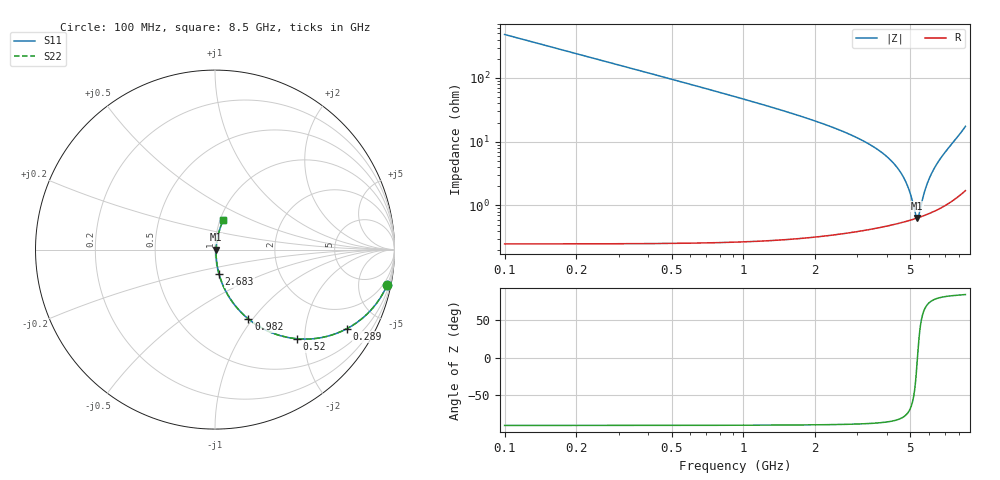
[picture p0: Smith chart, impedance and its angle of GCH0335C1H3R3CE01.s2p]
!Murata Part Number: GCH0335C1H3R3CE01
!These Parameters are Measured in Series Mode Connection
!Data Generated on Mar 13, 2026
!  o--ll--o
!Port1  Port2
!  o------o
!Operation Temp=25[degC], DC Bias Voltage=0[V]
!Freq. Start=100[MHz] Stop=9[GHz] 401[Steps]
# Hz S RI R 50
!Freq.(Hz) S11(Real) S11(Imag) S21(Real) S21(Imag) S12(Real) S12(Imag) S22(Real) S22(Imag)
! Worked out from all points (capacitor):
!   401 points, 100 MHz to 8.5 GHz, reference 50 ohm
!   read as one part in series: C = 3.3 pF near 142 MHz
!   lowest |Z| = 635 mohm at 5.35 GHz (marker M1)
!   series resonance near 5.354 GHz, so ESL is about 270 pH
!   S11 on the Smith chart (normalised r, x): 100 MHz: 1.00, -9.64; 289 MHz: 1.00, -3.33; 520 MHz: 1.01, -1.84; 982 MHz: 1.01, -0.95; 2.683 GHz: 1.01, -0.28; 8.5 GHz: 1.03, +0.35
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1e8  0.9587 -0.1988  0.0413 0.1988  0.0413 0.1988  0.9587 -0.1988
2.05e8  0.8464 -0.3601  0.1536 0.3601  0.1536 0.3601  0.8464 -0.3601
2.89e8  0.7345 -0.4409  0.2655 0.4409  0.2655 0.4409  0.7345 -0.4409
3.94e8  0.5972 -0.4894  0.4028 0.4894  0.4028 0.4894  0.5972 -0.4894
5.2e8  0.4583 -0.4969  0.5417 0.4969  0.5417 0.4969  0.4583 -0.4969
7.3e8  0.2976 -0.4552  0.7024 0.4552  0.7024 0.4552  0.2976 -0.4552
9.82e8  0.1863 -0.3866  0.8137 0.3866  0.8137 0.3866  0.1863 -0.3866
1.507e9  0.0834 -0.2717  0.9166 0.2717  0.9166 0.2717  0.0834 -0.2717
2.683e9  0.0223 -0.1352  0.9777 0.1352  0.9777 0.1352  0.0223 -0.1352
2.914e9  0.018 -0.1182  0.982 0.1182  0.982 0.1182  0.018 -0.1182
3.733e9  0.0094 -0.0698  0.9906 0.0698  0.9906 0.0698  0.0094 -0.0698
4.3e9  0.00689 -0.043  0.9931 0.043  0.9931 0.043  0.00689 -0.043
4.825e9  0.00605 -0.0209  0.994 0.0209  0.994 0.0209  0.00605 -0.0209
5.035e9  0.00603 -0.0125  0.994 0.0125  0.994 0.0125  0.00603 -0.0125
5.266e9  0.0062 -0.00341  0.9938 0.00341  0.9938 0.00341  0.0062 -0.00341
5.35e9  0.00631 -0.000148  0.9937 0.000148  0.9937 0.000148  0.00631 -0.000148
5.434e9  0.00645 0.00311  0.9936 -0.00311  0.9936 -0.00311  0.00645 0.00311
5.707e9  0.00707 0.0136  0.9929 -0.0136  0.9929 -0.0136  0.00707 0.0136
5.938e9  0.0078 0.0226  0.9922 -0.0226  0.9922 -0.0226  0.0078 0.0226
6.253e9  0.00916 0.035  0.9908 -0.035  0.9908 -0.035  0.00916 0.035
7.114e9  0.0155 0.0718  0.9845 -0.0718  0.9845 -0.0718  0.0155 0.0718
8.5e9  0.0445 0.1628  0.9555 -0.1628  0.9555 -0.1628  0.0445 0.1628
